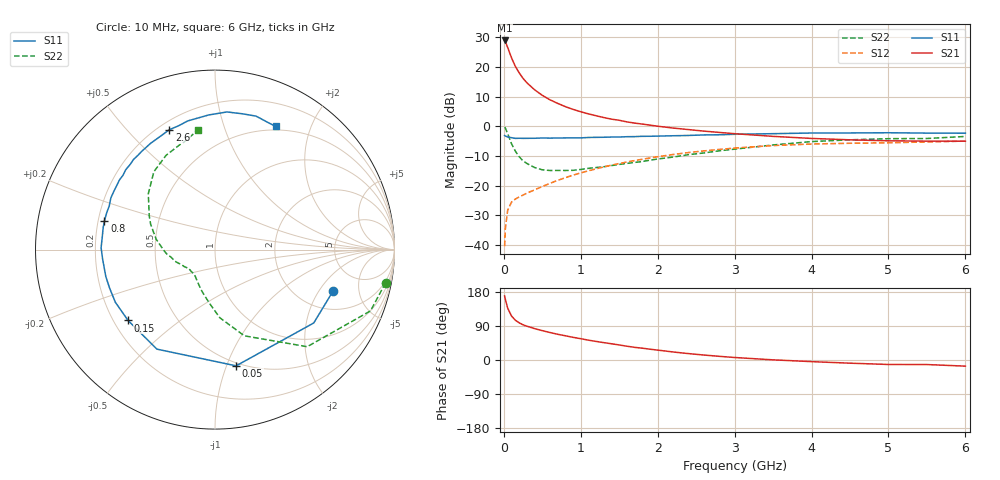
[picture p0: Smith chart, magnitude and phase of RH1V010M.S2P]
! SIEMENS Small Signal Semiconductors
! BFR106
! Si NPN RF Bipolar Junction Transistor in SOT23
! VCE = 1 V  IC = 10 mA
! Common Emitter S-Parameters:  August  1996
# GHz  S  MA  R  50
!  f  S11  S21  S12  S22
! GHz  MAG  ANG  MAG  ANG  MAG  ANG  MAG  ANG
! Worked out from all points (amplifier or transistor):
!   36 points, 10 MHz to 6 GHz, reference 50 ohm
!   highest |S21| = 29.0 dB at 10 MHz (marker M1)
!   |S21| within 3 dB of that: start of sweep to 59 MHz
!   unconditionally stable (mu >= 1): 460.5 MHz to 2.958 GHz; 3.993 GHz to end of sweep
!   at 250 MHz: K = 0.73, MSG = 19.7 dB, |S12| = -23.2 dB
!   at 1.4 GHz: K = 1.12, MAG = 5.6 dB, |S12| = -13.1 dB
!   at 6 GHz: K = 1.03, MAG = -1.1 dB, |S12| = -5.0 dB
!   S11 on the Smith chart (normalised r, x): 10 MHz: 3.05, -2.71; 50 MHz: 0.47, -1.08; 150 MHz: 0.26, -0.33; 800 MHz: 0.23, +0.12; 2.6 GHz: 0.24, +0.66; 6 GHz: 0.46, +1.51
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0.01  0.6977 -19.1  28.05 168.9  0.0095 82.8  0.9681 -11.0
0.02  0.6855 -36.6  26.85 159.9  0.0189 74.0  0.9315 -21.5
0.05  0.6582 -79.7  21.35 136.7  0.0385 55.9  0.7459 -46.5
0.1  0.6422 -120.3  14.27 116.1  0.0526 43.8  0.5074 -71.2
0.15  0.6248 -140.8  10.22 104.8  0.0593 40.0  0.3803 -86.0
0.2  0.628 -152.2  7.954 98.0  0.0644 40.6  0.3063 -95.0
0.25  0.6252 -160.1  6.423 92.8  0.0693 41.8  0.2603 -103.4
0.3  0.6266 -166.2  5.411 89.2  0.0745 44.0  0.2358 -109.3
0.4  0.6281 -174.9  4.126 82.8  0.0847 47.4  0.2015 -119.5
0.5  0.6347 179.1  3.327 77.5  0.0964 50.4  0.1846 -126.7
0.6  0.632 173.8  2.796 72.5  0.1091 52.3  0.1795 -131.6
0.8  0.6364 165.4  2.144 63.9  0.1358 54.6  0.1795 -141.2
0.9  0.6374 161.3  1.93 59.8  0.15 55.1  0.1808 -144.9
1.1  0.6478 153.6  1.619 52.3  0.1775 55.1  0.1953 -150.8
1.3  0.6533 147.1  1.403 45.8  0.2065 53.9  0.2079 -157.0
1.6  0.6673 138.2  1.186 36.4  0.2499 51.5  0.2365 -165.7
2.2  0.6923 121.2  0.934 21.2  0.3343 43.5  0.3024 176.3
2.6  0.7146 110.9  0.829 13.1  0.3845 37.3  0.3549 164.4
3.5  0.7509 92.7  0.676 0.4  0.4732 22.5  0.4844 140.1
4.5  0.772 78.5  0.591 -8.4  0.5172 7.3  0.5915 117.5
5.5  0.7676 67.7  0.562 -12.0  0.5441 -2.0  0.6225 106.3
6  0.7649 63.8  0.56 -16.2  0.5616 -8.6  0.6737 98.0
